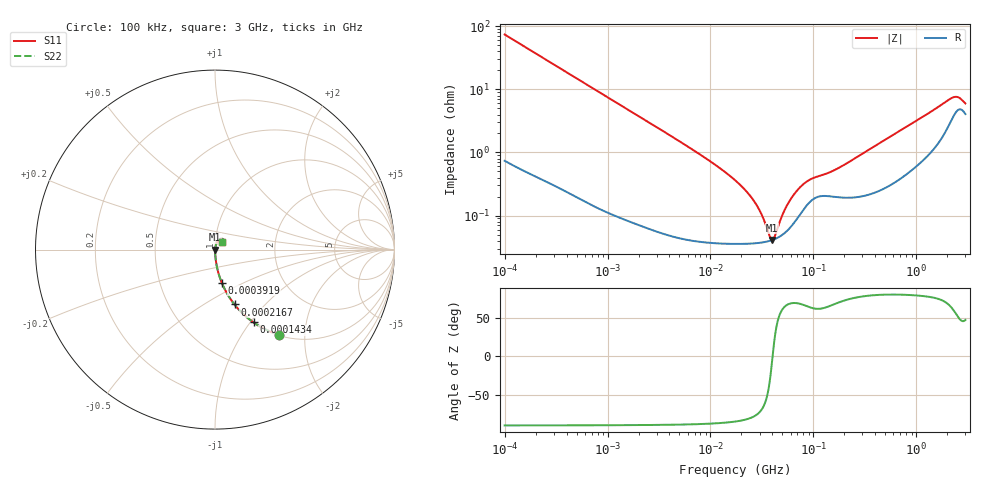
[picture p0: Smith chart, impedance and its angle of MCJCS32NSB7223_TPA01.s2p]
! MCJCS32NSB7223_TPA01  S-PARAMETER MODEL  ( Standard Model )
! Model Generated by TAIYO YUDEN Corporation (http://www.ty-top.com)
! Version 1.0
! TAIYO YUDEN Control No. 220601
! Copyright(c) 2015 TAIYO YUDEN CO.,LTD. All Rights Reserved.
! Product Description (link to TY-COMPAS)
! https://ds.yuden.co.jp/TYCOMPAS/or/detail?pn=MCJCS32NSB7223KTPA01&u=M
! Products Name : Multilayer Ceramic Capacitors
! Characteristics :
!  Capacitance : 0.022 [uF] , Rated Voltage : 630 [V] , TCC : X7R
!  Case Size : 3.2 x 2.5 / 0.126 x 0.098 [mm/inch] , Thickness : 1.9 / 0.075 [mm/inch]
!  (Conditions: Temperature = 25 [degC] , DC Bias Voltage = 0 [V])
! External Node Assignments :
!  1  o---| |---o  2
! GND o---------o GND
! Frequency Range : 100kHz  -  3GHz  [ 401 STEP ]
# MHZ S RI R 50
! Freq[MHz].  S11 Real  S11 Imag  S21 Real  S21 Imag  S12 Real  S12 Imag  S22 Real  S22 Imag
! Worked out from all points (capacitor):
!   401 points, 100 kHz to 3 GHz, reference 50 ohm
!   read as one part in series: C = 21.4 nF near 105.3 kHz
!   lowest |Z| = 41.2 mohm at 39.51 MHz (marker M1)
!   series resonance near 40.15 MHz, so ESL is about 730 pH
!   S11 on the Smith chart (normalised r, x): 100 kHz: 1.01, -1.49; 143.4 kHz: 1.01, -1.04; 216.7 kHz: 1.01, -0.69; 391.9 kHz: 1.00, -0.38; 3 GHz: 1.08, +0.09
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0.1  0.3571 -0.4742  0.6429 0.4742  0.6429 0.4742  0.3571 -0.4742
0.14345  0.2147 -0.4054  0.7853 0.4054  0.7853 0.4054  0.2147 -0.4054
0.216663  0.1089 -0.3059  0.8911 0.3059  0.8911 0.3059  0.1089 -0.3059
0.391939  0.0375 -0.1837  0.9625 0.1837  0.9625 0.1837  0.0375 -0.1837
0.562235  0.0192 -0.1309  0.9808 0.1309  0.9808 0.1309  0.0192 -0.1309
3.161081  0.00111 -0.0239  0.9989 0.0239  0.9989 0.0239  0.00111 -0.0239
9.574722  0.000427 -0.00754  0.9996 0.00754  0.9996 0.00754  0.000427 -0.00754
17.7727  0.000367 -0.00349  0.9996 0.00349  0.9996 0.00349  0.000367 -0.00349
27.54426  0.000366 -0.0015  0.9996 0.0015  0.9996 0.0015  0.000366 -0.0015
32.15051  0.000376 -0.000877  0.9996 0.000877  0.9996 0.000877  0.000376 -0.000877
37.52708  0.000396 -0.000267  0.9996 0.000267  0.9996 0.000267  0.000396 -0.000267
39.51212  0.000407 -6.29e-05  0.9996 6.29e-05  0.9996 6.29e-05  0.000407 -6.29e-05
41.60216  0.000419 0.000142  0.9996 -0.000142  0.9996 -0.000142  0.000419 0.000142
51.12795  0.00051 0.000986  0.9995 -0.000986  0.9995 -0.000986  0.00051 0.000986
61.23616  0.000683 0.00177  0.9993 -0.00177  0.9993 -0.00177  0.000683 0.00177
77.22239  0.00115 0.00276  0.9989 -0.00276  0.9989 -0.00276  0.00115 0.00276
97.38194  0.00178 0.00343  0.9982 -0.00343  0.9982 -0.00343  0.00178 0.00343
176.1623  0.00197 0.00532  0.998 -0.00532  0.998 -0.00532  0.00197 0.00532
547.5153  0.00325 0.0171  0.9967 -0.0171  0.9967 -0.0171  0.00325 0.0171
2201.951  0.0356 0.0608  0.9644 -0.0608  0.9644 -0.0608  0.0356 0.0608
2504.792  0.0472 0.0548  0.9528 -0.0548  0.9528 -0.0548  0.0472 0.0548
3000  0.0408 0.0406  0.9592 -0.0406  0.9592 -0.0406  0.0408 0.0406
